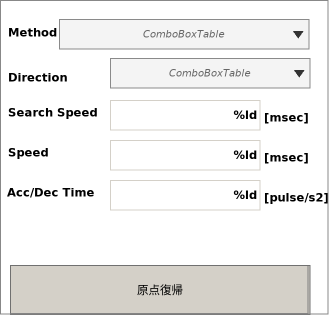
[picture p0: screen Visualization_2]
VISUALIZATION Visualization_2  // 329x315
    Label (5,20 90x25), "Method"
    Label (5,65 90x25), "Direction"
    Textfield (110,100 150x30), "%ld", text variable: move_prg.search_speed
        OnMouseClick: write the text variable via Default, min 1, max 500000, format 1000
    Label (5,100 90x25), "Search Speed"
    Label (261,105 50x25), "[msec]"
    Textfield (110,140 150x30), "%ld", text variable: move_prg.homing_speed
        OnMouseClick: write the text variable via Default, min 1, max 2500000, format 10000
    Label (5,140 90x25), "Speed"
    Label (261,145 50x25), "[msec]"
    Textfield (110,180 150x30), "%ld", text variable: main.profile_acceleration
        OnMouseClick: write the text variable via Default, min 1000, max 1000000000, format 1000000
    Label (4,180 90x25), "Acc/Dec Time"
    Label (261,185 68x25), "[pulse/s2]"
    Button (10,265 300x50), "原点復帰"
        tap move_prg.home_sw
    ComboBoxTable (59,19 250x30), variable: move_prg.org_method, data array: move_prg.meshod_table
        p3854506369: move_prg.meshod_table[INDEX]
    ComboBoxTable (110,58 200x30), variable: move_prg.org_dir, data array: move_prg.dir_table
        p3854506369: move_prg.dir_table[INDEX]
END_VISUALIZATION
